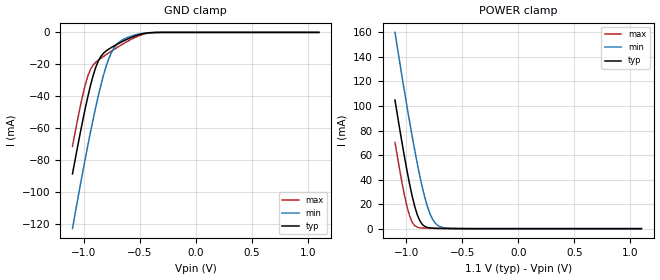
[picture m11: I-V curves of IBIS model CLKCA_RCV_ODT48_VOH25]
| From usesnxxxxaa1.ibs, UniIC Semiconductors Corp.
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|   Model CLKCA_RCV_ODT48_VOH25
[Model] CLKCA_RCV_ODT48_VOH25
Model_type Input
Polarity   Non-Inverting
Vinl =  0.113V
Vinh =  0.253V
C_comp   0.852pF   0.835pF   0.861pF
[Model Spec]
Vinh   0.253V   0.247V   0.265V
Vinl   0.113V   0.107V   0.125V
[Add Submodel]
|  Submodel_name   Mode
ODT48_VOH25   Non-Driving
[Temperature Range]   25.000   0.125k   -40.000
[Voltage Range]   1.100V   1.060V   1.170V
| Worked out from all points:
|   GND clamp passes 1 mA (typ) near -0.48 V on its own axis
|   POWER clamp passes 1 mA (typ) near -0.81 V on its own axis
[GND_clamp]
|Voltage   I(typ)   I(min)   I(max)
-1.1V     -88.79mA   -123.1mA   -71.48mA
-1.031V   -63.25mA   -96.13mA   -46.59mA
-985mV    -47.4mA    -78.91mA   -32.65mA
-939mV    -33.23mA   -62.49mA   -23.22mA
-893mV    -22.03mA   -47.12mA   -18.8mA
-847mV    -15.14mA   -33.24mA   -16.26mA
-778mV    -10.55mA   -16.86mA   -12.94mA
-732mV    -8.616mA   -10.04mA   -10.83mA
-686mV    -6.865mA   -6.259mA   -8.795mA
-548mV    -2.421mA   -1.734mA   -3.398mA
-387mV    -126.8uA   -122.3uA   -186.4uA
1.1V      0A         0A         0A
[POWER_clamp]
|Voltage   I(typ)   I(min)   I(max)
-1.1V     104.8mA    160mA      70.36mA
-1.039V   71.02mA    125.1mA    38.37mA
-993mV    47.41mA    99.76mA    18.16mA
-970mV    36.61mA    87.48mA    10.56mA
-947mV    26.77mA    75.56mA    5.326mA
-901mV    11.35mA    53.11mA    1.208mA
-855mV    3.329mA    33.33mA    538.3uA
-809mV    890.1uA    17.63mA    399uA
-763mV    354.9uA    7.445mA    322.9uA
-717mV    219.7uA    2.583mA    258.1uA
-556mV    65.25uA    87.5uA     81.64uA
1.1V      0A         0A         1.291pA
